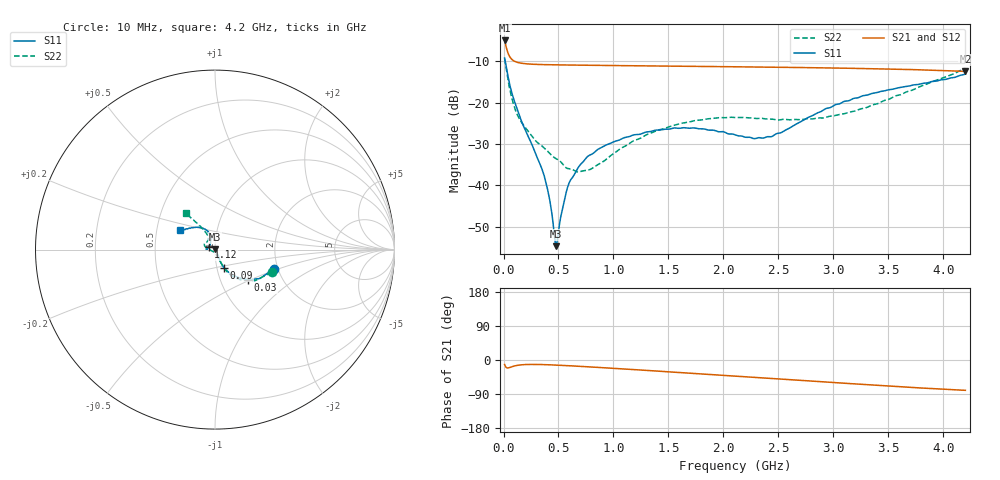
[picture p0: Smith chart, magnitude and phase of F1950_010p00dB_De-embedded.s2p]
! Integrated Device Technology
! Corporate Headquarters
! 6024 Silver Creek Valley Road
! San Jose, CA 95138  USA
! Phone:  1-408-284-8200
! Toll Free:  1-800-223-1366
! Webpage:  http://www.idt.com/
! Timing and RF Division
! 515 Groton Road, Suite 102
! Westford, MA 01886-6024
! Device:  F1950
! Description: 7-bit 0.25 dB Digital Step Attenuator
! Frequency:  150.0 -  4000.00 MHz
! Package:  4x4 mm Thin QFN Plastic Package: 24 pin
! Ports:  2 RF, 12 DC
!  Pin  1  = D0
!  Pin  2  = VDD
!  Pin  3  = Vmode
!  Pin  4  = GND
!  Pin  5  = RF1  =  Port 1
!  Pin  6  = GND
!  Pin  7  = GND
!  Pin  8  = GND
!  Pin  9  = GND
!  Pin 10  = GND
!  Pin 11  = GND
!  Pin 12  = GND
!  Pin 13  = GND
!  Pin 14  = RF2  =  Port 2
!  Pin 15  = GND
!  Pin 16  = LE
!  Pin 17  = CLK
!  Pin 18  = DATE
!  Pin 19  = D6
!  Pin 20  = D5
!  Pin 21  = D4
!  Pin 22  = D3
!  Pin 23  = D2
!  Pin 24  = D1
! State:  40
! Atten State:  10.00 dB
! Voltage:  +5.00 Volts
! Current:  Not Measured mA
! Data:  The device was measured on a the F195X evaluation board which has
!  individual transmission lines to the RF pins.  Data was collected
!  using a calibrated network analyzer.  The evaluation board was
!  de-embedded using a TRL calibration technique.
!  The reference plane is the edge of the package pin.
! Misc:  Board 2019
!  Action Tracker AT0250
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# GHz S dB R 50
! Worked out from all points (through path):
!   420 points, 10 MHz to 4.2 GHz, reference 50 ohm
!   highest |S21| = -4.96 dB at 10 MHz (marker M1); lowest = -12.4 dB at 4.2 GHz (marker M2)
!   group delay of S21, straight-line fit = 49 ps
!   lowest |S11| = -54.7 dB at 480 MHz (marker M3), VSWR 1.00, Z = 50.1 + j0.125 ohm
!   |S11| at or under -10 dB: 15.97 MHz to end of sweep
!   |S22| runs from -36.7 to -9.3 dB; largest |S21 - S12| = 0.00039
!   S11 on the Smith chart (normalised r, x): 10 MHz: 1.91, -0.46; 30 MHz: 1.35, -0.49; 90 MHz: 1.08, -0.22; 1.12 GHz: 0.93, +0.03; 4.2 GHz: 0.66, +0.15
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0.01  -9.21 -18.0  -4.96 -11.8  -4.96 -11.8  -9.35 -21.7
0.03  -12.04 -42.3  -7.10 -20.7  -7.10 -20.7  -12.77 -48.4
0.05  -14.82 -53.6  -8.57 -20.4  -8.57 -20.4  -15.83 -58.8
0.09  -18.90 -63.4  -9.83 -16.4  -9.83 -16.4  -20.29 -64.4
0.17  -24.89 -65.2  -10.49 -12.5  -10.49 -12.6  -25.01 -68.2
0.36  -36.87 -52.9  -10.80 -12.1  -10.79 -12.1  -30.71 -74.0
0.41  -42.11 -47.2  -10.82 -12.6  -10.82 -12.6  -31.97 -75.0
0.46  -51.51 -13.9  -10.85 -13.2  -10.85 -13.2  -33.23 -81.4
0.48  -54.68 42.7  -10.86 -13.4  -10.86 -13.5  -33.56 -84.2
0.49  -53.15 71.4  -10.86 -13.6  -10.86 -13.6  -33.70 -85.2
0.59  -39.86 123.2  -10.90 -15.0  -10.90 -15.1  -35.92 -100.0
0.71  -34.68 133.3  -10.93 -17.0  -10.93 -17.0  -36.56 -123.9
0.87  -31.10 143.0  -10.98 -19.7  -10.98 -19.7  -34.80 -155.1
1.12  -28.34 156.7  -11.06 -24.1  -11.06 -24.1  -30.30 -179.4
1.41  -26.62 169.3  -11.13 -29.4  -11.13 -29.4  -26.60 169.6
1.73  -26.10 177.3  -11.22 -35.3  -11.22 -35.3  -24.38 161.2
2.11  -27.83 170.0  -11.32 -42.5  -11.32 -42.5  -23.59 151.4
2.43  -28.23 135.8  -11.42 -48.5  -11.42 -48.5  -23.96 141.0
2.81  -23.12 109.4  -11.54 -55.8  -11.54 -55.8  -23.92 125.3
3.1  -19.67 110.8  -11.66 -61.3  -11.66 -61.4  -22.66 119.2
3.51  -16.84 122.1  -11.87 -68.9  -11.86 -68.9  -19.12 118.8
4.2  -13.10 151.0  -12.44 -80.0  -12.44 -80.1  -11.71 128.9
